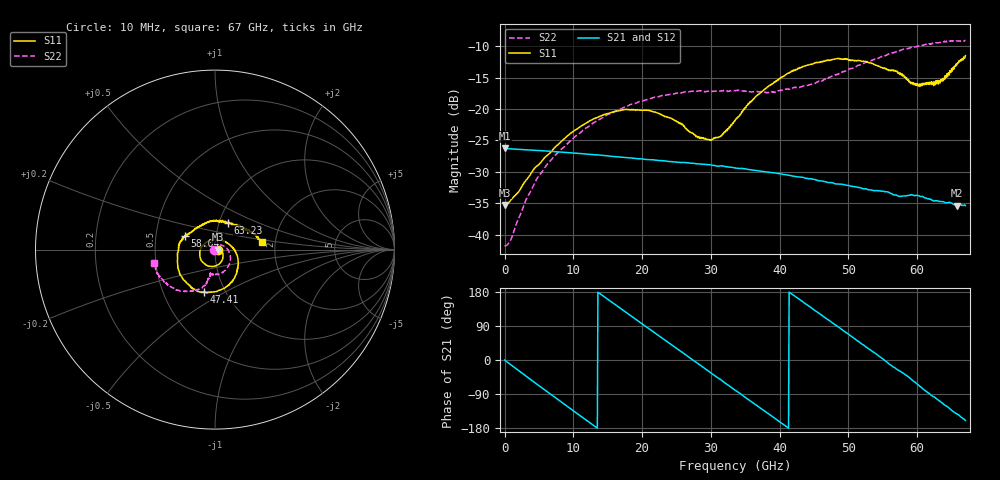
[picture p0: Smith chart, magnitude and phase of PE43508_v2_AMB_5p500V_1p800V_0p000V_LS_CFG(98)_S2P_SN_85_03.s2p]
!Keysight Technologies,N5227A,US51270237,A.10.43.00
!Date: Wednesday, August 22, 2018 17:16:54
!Correction: S11(Full 2 Port(1,3))
!S31(Full 2 Port(1,3))
!S13(Full 2 Port(1,3))
!S33(Full 2 Port(1,3))
!S2P File: Measurements: S11, S31, S13, S33:
# Hz S  dB  R 50
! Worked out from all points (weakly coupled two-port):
!   801 points, 10 MHz to 67 GHz, reference 50 ohm
!   highest |S21| = -26.26 dB at 10 MHz (marker M1); lowest = -35.4 dB at 65.83 GHz (marker M2)
!   lowest |S11| = -35.3 dB at 93.74 MHz (marker M3), VSWR 1.04, Z = 51.8 + j0.0154 ohm
!   |S11| at or under -10 dB: start of sweep to end of sweep
!   |S22| runs from -41.8 to -9.1 dB; largest |S21 - S12| = 0.00025
!   S11 on the Smith chart (normalised r, x): 10 MHz: 1.04, -0.00; 47.41 GHz: 0.79, -0.40; 58.04 GHz: 0.70, +0.11; 63.23 GHz: 1.10, +0.34; 67 GHz: 1.70, +0.15
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1e7  -35.19 -1.1  -26.26 -0.3  -26.26 -0.2  -41.80 -179.2
9.37375e7  -35.27 0.5  -26.28 -1.4  -26.29 -1.4  -41.73 174.8
9.311125e8  -34.45 3.9  -26.34 -13.0  -26.34 -13.0  -40.74 134.6
3.108288e9  -31.31 2.1  -26.48 -42.5  -26.48 -42.5  -34.45 80.7
4.866775e9  -28.92 -7.1  -26.59 -66.0  -26.60 -66.0  -30.78 59.9
7.3789e9  -26.02 -27.7  -26.78 -99.4  -26.78 -99.4  -27.34 36.7
1.123082e10  -22.63 -60.1  -27.10 -150.2  -27.10 -150.2  -23.56 5.2
1.74274e10  -20.10 -111.4  -27.68 128.9  -27.68 128.9  -19.69 -34.4
2.236791e10  -20.68 -155.1  -28.18 64.8  -28.17 64.7  -18.04 -60.0
2.973681e10  -24.90 96.4  -28.86 -30.4  -28.86 -30.5  -17.13 -87.3
3.14953e10  -24.22 59.8  -29.03 -52.9  -29.03 -52.9  -17.16 -92.5
3.3505e10  -21.91 24.2  -29.36 -79.5  -29.37 -79.5  -17.08 -96.9
3.88642e10  -16.10 -35.4  -30.10 -148.3  -30.11 -148.2  -17.31 -101.2
4.472582e10  -12.86 -83.9  -31.13 135.9  -31.11 135.9  -16.07 -101.6
4.740542e10  -12.22 -104.7  -31.68 101.7  -31.64 101.6  -14.89 -103.8
5.234594e10  -12.41 -144.1  -32.68 37.4  -32.64 37.2  -12.67 -110.8
5.586291e10  -13.90 -179.5  -33.25 -9.8  -33.22 -10.2  -11.25 -121.6
5.804009e10  -14.61 155.4  -33.80 -35.8  -33.81 -36.1  -10.47 -129.3
6.004979e10  -16.00 122.1  -33.71 -64.2  -33.73 -64.6  -10.08 -137.0
6.323181e10  -15.55 64.4  -34.67 -108.0  -34.72 -108.7  -9.43 -150.7
6.582768e10  -12.74 24.1  -35.36 -142.8  -35.46 -143.2  -9.20 -161.3
6.7e10  -11.52 8.8  -35.36 -159.7  -35.44 -159.6  -9.14 -167.9
